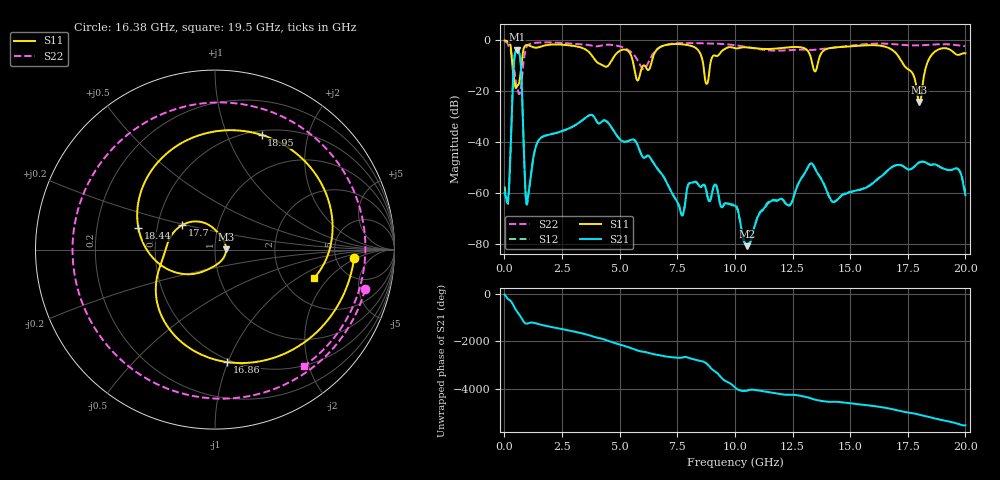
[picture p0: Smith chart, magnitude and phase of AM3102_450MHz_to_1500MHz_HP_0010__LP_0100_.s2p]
!Agilent Technologies,E8364B,MY43040894,A.07.50.67
!Agilent E8364B: A.07.50.67
!Date: Thursday, January 11, 2018 05:24:42
!Correction: S11(Full 2 Port(1,2))
!S21(Full 2 Port(1,2))
!S12(Full 2 Port(1,2))
!S22(Full 2 Port(1,2))
!S2P File: Measurements: S11, S21, S12, S22:
# Hz S  dB  R 50
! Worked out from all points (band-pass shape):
!   1601 points, 10 MHz to 20 GHz, reference 50 ohm
!   highest |S21| = -3.71 dB at 547.2 MHz (marker M1); lowest = -80.7 dB at 10.54 GHz (marker M2)
!   |S21| within 3 dB of the highest: 437.3 MHz to 683.2 MHz (245.9 MHz wide, 43.9 % of centre)
!   lowest |S11| = -24.2 dB at 18 GHz (marker M3), VSWR 1.13, Z = 56.6 + j0.122 ohm
!   |S11| at or under -10 dB: 349.5 MHz to 737.2 MHz (387.7 MHz wide, 71.4 % of centre); 5.614 GHz to 6.015 GHz (401.1 MHz wide, 6.9 % of centre); 17.35 GHz to 18.31 GHz (951.6 MHz wide, 5.34 % of centre)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
!   |S22| runs from -21.1 to -0.3 dB; largest |S21 - S12| = 0.002
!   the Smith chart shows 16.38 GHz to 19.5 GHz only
!   S11 on the Smith chart (normalised r, x): 16.38 GHz: 7.48, -1.83; 16.86 GHz: 0.48, -0.99; 17.7 GHz: 0.67, +0.19; 18.44 GHz: 0.39, +0.12; 18.95 GHz: 0.55, +1.34; 19.5 GHz: 2.99, -1.40
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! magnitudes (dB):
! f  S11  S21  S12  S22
! 10 MHz  -0.1  -59.8  -57.2  -0.3
! 172.4 MHz  -0.6  -61.3  -62.9  -2.0
! 547.2 MHz  -18.2  -3.7  -3.7  -18.4
! 997 MHz  -1.9  -63.6  -63.6  -2.1
! 1.509 GHz  -2.7  -38.9  -38.9  -0.9
! 3.346 GHz  -2.9  -31.6  -31.6  -1.5
! 6.682 GHz  -3.1  -50.9  -50.8  -3.1
! 7.694 GHz  -1.5  -68.5  -68.5  -1.1
! 8.781 GHz  -17.1  -59.8  -60.0  -1.2
! 10.01 GHz  -3.1  -64.8  -64.3  -1.9
! 10.54 GHz  -2.8  -80.7  -80.2  -2.7
! 13.34 GHz  -8.4  -48.3  -48.3  -3.8
! 14.28 GHz  -2.8  -63.3  -63.4  -2.9
! 16.38 GHz  -2.2  -53.2  -53.0  -1.3
! 16.68 GHz  -3.0  -50.7  -50.6  -1.4
! 16.86 GHz  -4.0  -49.4  -49.5  -1.5
! 17.7 GHz  -12.8  -50.2  -50.2  -2.0
! 18 GHz  -24.2  -47.9  -47.8  -2.0
! 18.44 GHz  -7.1  -48.7  -48.7  -1.8
! 18.95 GHz  -3.2  -49.9  -49.9  -1.5
! 19.5 GHz  -4.8  -50.5  -50.5  -1.8
! 20 GHz  -5.1  -60.7  -59.3  -2.3
